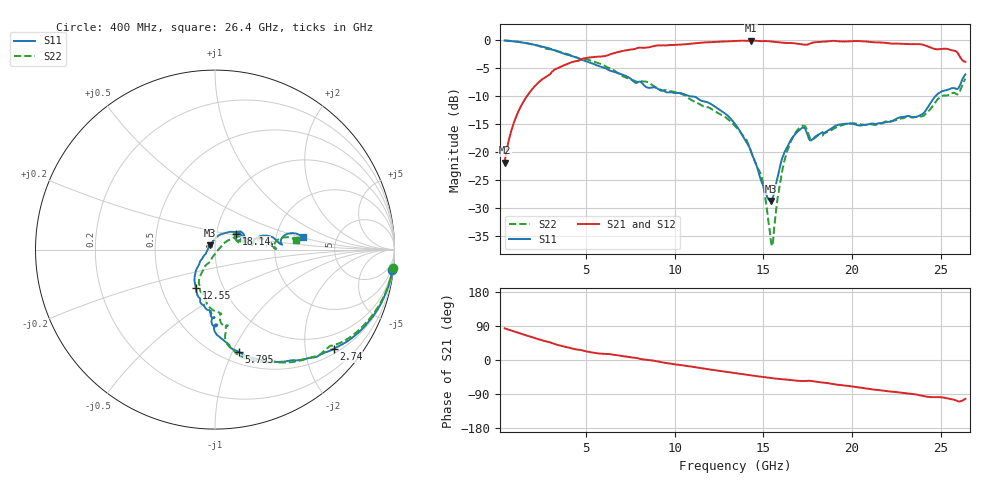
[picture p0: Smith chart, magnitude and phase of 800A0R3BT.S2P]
!  American Technical Ceramics  Date:  12/17/08
!  One Norden Lane
!  Huntington Station,  NY.  11746-2102
!  Tel:  (631) 622-4700  Fax:  (631) 622-4748
!  Part Number  800A0R3BT
!  Description: Broardband capacitor  Mounting Orientation: Vertical
!  Application:
# GHZ S DB R 50
! Freq  |S11|  S11 Ph  |S21|  S21 Ph  |S12|  S12 Ph  |S22|  S22 Ph
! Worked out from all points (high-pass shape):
!   401 points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, 400 MHz to 26.4 GHz, reference 50 ohm
!   highest |S21| = -0.05 dB at 14.31 GHz (marker M1); lowest = -21.8 dB at 400 MHz (marker M2)
!   |S21| within 3 dB of the highest: 5.232 GHz to 26.12 GHz (20.88 GHz wide, 133 % of centre)
!   lowest |S11| = -28.7 dB at 15.41 GHz (marker M3), VSWR 1.08, Z = 47.2 + j2.26 ohm
!   |S11| at or under -10 dB: 10.85 GHz to 24.7 GHz (13.85 GHz wide, 77.9 % of centre)
!   |S22| runs from -36.7 to 0.0 dB; largest |S21 - S12| = 0.0018
!   S11 on the Smith chart (normalised r, x): 400 MHz: 1, -17; 2.74 GHz: 0.61, -2.63; 5.795 GHz: 0.61, -1.05; 12.55 GHz: 0.74, -0.34; 18.14 GHz: 1.24, +0.22; 26.4 GHz: 2.87, +0.52
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0.4  -0.04 -6.7  -21.83 83.5  -21.83 83.5  -0.02 -5.8
1.31  -0.34 -21.0  -11.83 69.5  -11.83 69.5  -0.32 -19.1
2.74  -1.29 -39.9  -6.51 49.1  -6.51 49.0  -1.48 -39.4
4.755  -3.48 -66.9  -3.34 25.8  -3.34 25.8  -3.28 -63.5
5.795  -4.68 -77.0  -2.90 16.8  -2.89 16.8  -4.18 -75.5
9.11  -8.78 -93.9  -0.91 -4.8  -0.91 -4.8  -8.65 -85.6
12.555  -12.45 -116.5  -0.23 -28.9  -0.23 -28.9  -13.18 -113.1
13.4  -14.93 -128.4  -0.12 -34.5  -0.12 -34.5  -15.28 -119.1
14.31  -19.89 -142.7  -0.05 -40.4  -0.05 -40.5  -19.87 -120.2
14.895  -25.22 -156.8  -0.15 -44.2  -0.15 -44.2  -24.30 -109.6
15.415  -28.68 139.5  -0.19 -47.5  -0.19 -47.6  -35.67 -62.5
15.545  -27.95 119.6  -0.24 -48.3  -0.24 -48.3  -35.96 -11.9
16.13  -20.48 66.3  -0.43 -51.0  -0.43 -51.1  -22.30 35.7
16.585  -17.62 49.0  -0.48 -53.0  -0.48 -53.1  -17.80 32.5
17.235  -15.56 29.9  -0.74 -55.5  -0.74 -55.5  -15.22 20.9
17.755  -17.73 31.6  -0.43 -55.6  -0.43 -55.6  -17.75 26.2
18.145  -16.77 36.9  -0.29 -58.5  -0.30 -58.5  -16.92 37.9
22.11  -14.54 16.9  -0.54 -82.9  -0.54 -83.0  -14.40 14.2
23.865  -13.33 10.8  -0.70 -93.5  -0.69 -93.5  -13.58 8.1
25.295  -8.92 5.7  -1.49 -100.4  -1.49 -100.4  -9.84 2.1
26.01  -8.54 9.2  -2.48 -109.2  -2.48 -109.3  -9.56 5.8
26.4  -6.07 7.8  -3.82 -102.5  -3.82 -102.5  -6.86 6.7
